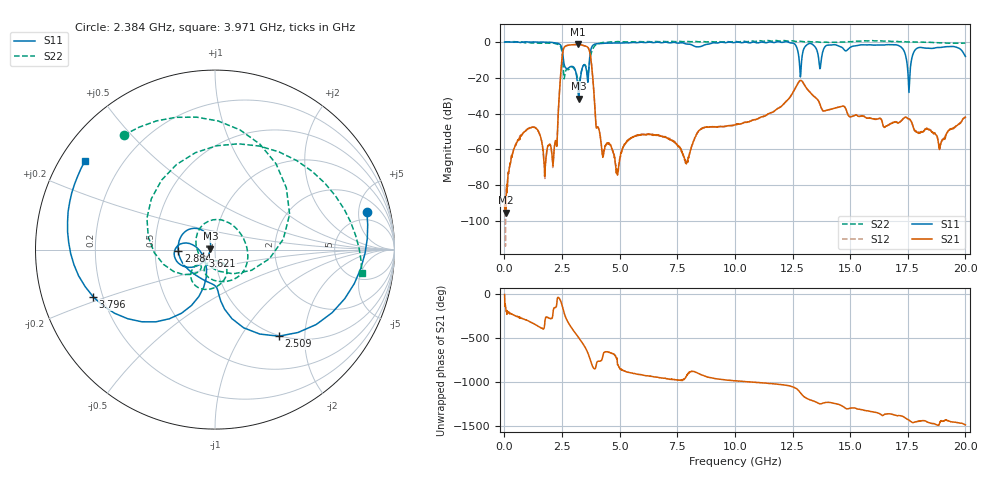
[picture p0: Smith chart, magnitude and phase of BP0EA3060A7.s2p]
! 9/17/2020 12:46:50 PM
! C:\ANRITSUVNA\DATA\MLO\SAMPLES\RAYTHEOM BP\17366_20GH_91720 .S2P
! CHANNEL.1
! TR.MEASUREMENT
! CORRECTED.DATA
# GHZ S RI R 50.0
! FREQ.GHZ  S11RE  S11IM  S31RE  S31IM  S13RE  S13IM  S33RE  S33IM
!; PortSelection: Port_13
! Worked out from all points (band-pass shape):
!   1601 points, 10 MHz to 20 GHz, reference 50 ohm
!   highest |S21| = -1.49 dB at 3.196 GHz (marker M1); lowest = -95.2 dB at 72.47 MHz (marker M2)
!   |S21| within 3 dB of the highest: 2.553 GHz to 3.677 GHz (1.123 GHz wide, 36.1 % of centre)
!   lowest |S11| = -31.6 dB at 3.221 GHz (marker M3), VSWR 1.05, Z = 47.5 + j0.552 ohm
!   |S11| at or under -10 dB: 2.564 GHz to 3.692 GHz (1.128 GHz wide, 36.1 % of centre); 12.79 GHz to 12.9 GHz (111.9 MHz wide, 0.871 % of centre); 17.44 GHz to 17.66 GHz (219 MHz wide, 1.25 % of centre)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
!   |S22| runs from -24.2 to 0.7 dB; largest |S21 - S12| = 0.0031
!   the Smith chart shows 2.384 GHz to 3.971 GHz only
!   S11 on the Smith chart (normalised r, x): 2.384 GHz: 3.51, +6.19; 2.509 GHz: 0.99, -1.49; 2.884 GHz: 0.66, -0.01; 3.621 GHz: 0.87, -0.06; 3.796 GHz: 0.16, -0.18; 3.971 GHz: 0.07, +0.31
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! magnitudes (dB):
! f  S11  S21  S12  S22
! 10 MHz  -0.2  -91.1  -92.7  0.0
! 72.47 MHz  0.0  -95.2  -86.3  -0.1
! 1.01 GHz  -0.1  -48.6  -48.5  -0.4
! 2.171 GHz  -0.5  -58.1  -58.2  -0.9
! 2.384 GHz  -1.2  -29.1  -29.0  -1.8
! 2.509 GHz  -4.5  -8.2  -8.2  -6.7
! 2.884 GHz  -13.8  -1.7  -1.7  -14.2
! 3.196 GHz  -27.5  -1.5  -1.5  -22.6
! 3.221 GHz  -31.6  -1.5  -1.5  -24.1
! 3.346 GHz  -16.4  -1.8  -1.8  -16.2
! 3.621 GHz  -22.5  -3.1  -3.1  -18.6
! 3.796 GHz  -2.8  -14.5  -14.4  -5.2
! 3.971 GHz  -1.1  -45.9  -45.9  -1.6
! 4.895 GHz  -0.7  -72.5  -74.3  0.1
! 6.682 GHz  -0.2  -52.0  -51.9  0.1
! 7.894 GHz  -1.2  -68.1  -66.9  0.2
! 10.01 GHz  -0.3  -46.3  -46.4  0.2
! 13.34 GHz  -1.2  -29.3  -29.3  -0.1
! 16.68 GHz  -1.6  -46.3  -46.3  0.4
! 17.55 GHz  -28.2  -43.0  -43.0  -0.1
! 18.91 GHz  -3.1  -57.1  -57.3  -0.6
! 20 GHz  -8.1  -42.1  -42.3  -0.7
